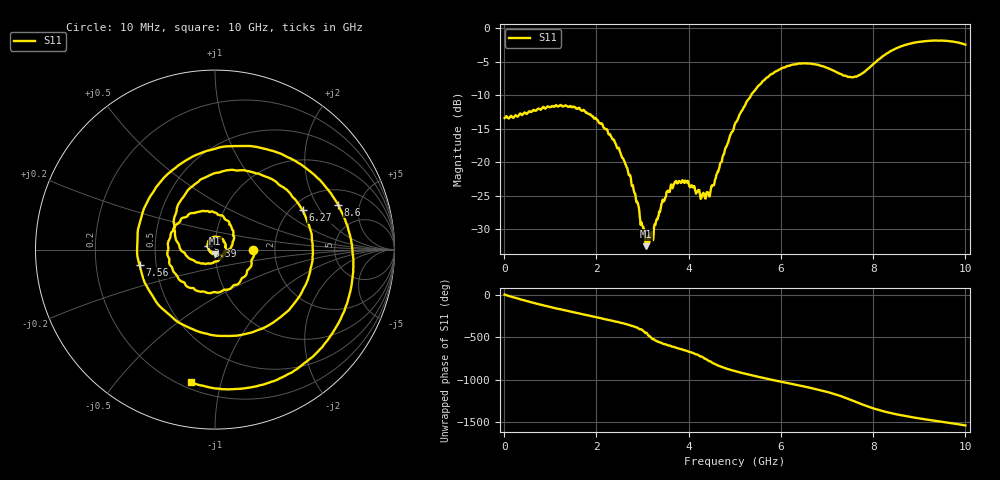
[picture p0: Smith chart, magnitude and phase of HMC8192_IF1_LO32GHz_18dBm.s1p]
! Analog Devices, Inc.
! 1 Analog Way
! Wilmington, MA 01887
! http://www.analog.com
! Date:  2021-09-17 NN
! Board Name:  EVALHMC8192LG Revision A with HMC8192LG installed
! File Description:  S-Parameters for evaluation board without connectors or board loss de-embedded
! File Generation:  Calibrated Network Analyzer
! Chip Part Number:  HMC8192
! Chip Description:  Wideband IQ Mixer
! Chip Frequency:  20 to 42 GHz
! Chip Package:  LGA_CAV, 4 x 4 x 1.55 mm
! Chip State:
!  Temperature:  25C
!  LO Frequency:  32GHz
!  LO Power:  18dBm
! Note:
!  Analog Devices supplies this data as a sample of measured data at the evaluation board
!  ports for this product.  Your particular data for this product may vary.
!  Analog Devices reserves the right to change this data at anytime.
!  All lines below in this file are as is from the Network Analyzer.
!Keysight Technologies,N5245A,MY49151104,A.10.65.16
!Date: Tuesday, September 14, 2021 12:21:39
!Correction: S22(Full 2 Port(1,2))
!S1P File: Measurement: S22:
# Hz S  dB  R 50
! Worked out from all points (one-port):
!   1000 points, 10 MHz to 10 GHz, reference 50 ohm
!   lowest |S11| = -32.5 dB at 3.07 GHz (marker M1), VSWR 1.05, Z = 49.8 - j2.35 ohm
!   |S11| at or under -10 dB: start of sweep to 5.355 GHz
!   S11 on the Smith chart (normalised r, x): 10 MHz: 1.54, -0.00; 3.39 GHz: 0.92, +0.03; 6.27 GHz: 2.30, +1.41; 7.56 GHz: 0.40, -0.09; 8.6 GHz: 2.88, +3.11; 10 GHz: 0.24, -0.81
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1e7  -13.41 -0.4
6e8  -12.47 -92.5
1.26e9  -11.67 -179.9
1.87e9  -12.89 108.4
2.51e9  -18.47 29.0
3.07e9  -32.54 -92.8
3.19e9  -30.99 -150.2
3.39e9  -26.97 155.8
3.76e9  -23.16 89.0
4.41e9  -24.78 -52.5
5.01e9  -14.25 178.5
5.37e9  -9.81 129.7
5.74e9  -7.16 84.5
6.26e9  -5.46 25.2
6.27e9  -5.44 24.1
6.65e9  -5.31 -19.5
7.03e9  -6.01 -69.8
7.27e9  -6.80 -109.3
7.51e9  -7.31 -157.5
7.56e9  -7.35 -168.4
7.79e9  -6.63 141.6
8.08e9  -4.91 88.0
8.31e9  -3.74 54.2
8.6e9  -2.73 20.1
8.76e9  -2.38 4.1
9.09e9  -1.97 -25.2
9.46e9  -1.87 -54.9
1e10  -2.47 -100.4
